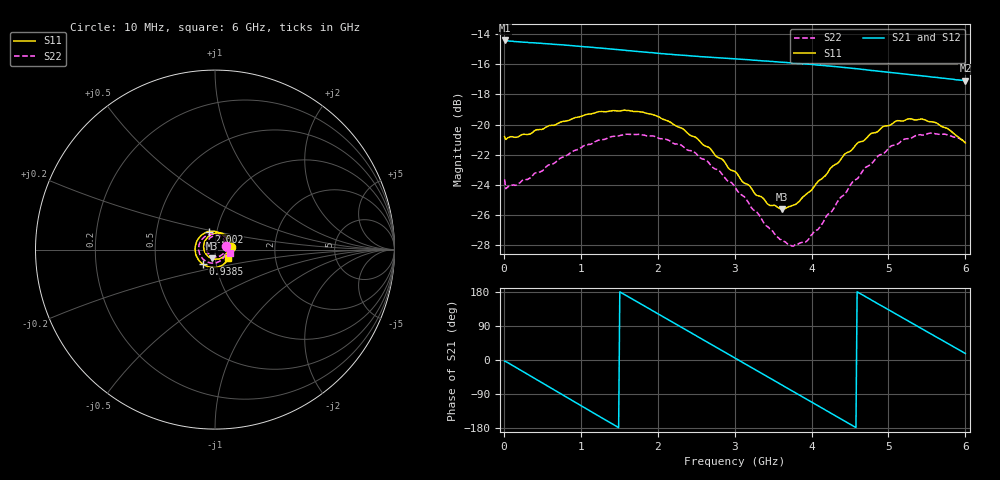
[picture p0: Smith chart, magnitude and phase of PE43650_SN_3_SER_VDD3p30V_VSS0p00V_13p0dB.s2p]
!Keysight Technologies,N5245B,MY57181451,A.13.50.07
!Date: Tuesday, May 07, 2019 08:00:11
!Correction: S11(Full 2 Port(1,2))
!S21(Full 2 Port(1,2))
!S12(Full 2 Port(1,2))
!S22(Full 2 Port(1,2))
!S2P File: Measurements: S11, S21, S12, S22:
# Hz S  dB  R 50
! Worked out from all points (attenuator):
!   401 points, 10 MHz to 6 GHz, reference 50 ohm
!   highest |S21| = -14.42 dB at 10 MHz (marker M1); lowest = -17.1 dB at 6 GHz (marker M2)
!   lowest |S11| = -25.6 dB at 3.619 GHz (marker M3), VSWR 1.11, Z = 47.9 - j4.67 ohm
!   |S11| at or under -10 dB: start of sweep to end of sweep
!   |S22| runs from -28.1 to -20.6 dB; largest |S21 - S12| = 0.0014
!   S11 on the Smith chart (normalised r, x): 10 MHz: 1.20, +0.03; 938.5 MHz: 0.86, -0.14; 2.002 GHz: 0.92, +0.19; 6 GHz: 1.15, -0.11
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1e7  -20.81 9.0  -14.42 -3.3  -14.48 -3.4  -23.64 16.9
2.496e8  -20.66 -37.1  -14.54 -30.7  -14.58 -30.7  -23.69 -36.8
5.1915e8  -20.28 -75.2  -14.63 -63.0  -14.67 -63.0  -22.98 -75.5
9.3845e8  -19.53 -129.5  -14.79 -113.0  -14.84 -113.0  -21.70 -127.6
1.013325e9  -19.45 -138.8  -14.82 -121.8  -14.87 -121.9  -21.50 -136.6
1.2679e9  -19.14 -168.7  -14.93 -152.0  -14.99 -151.9  -21.02 -164.6
1.492525e9  -19.10 165.3  -15.03 -178.4  -15.10 -178.4  -20.76 171.4
1.732125e9  -19.13 138.5  -15.15 153.5  -15.21 153.5  -20.66 146.6
2.001675e9  -19.47 109.0  -15.27 122.0  -15.33 122.0  -20.89 119.5
2.01665e9  -19.50 107.3  -15.28 120.2  -15.33 120.3  -20.91 117.9
2.241275e9  -20.10 82.1  -15.37 94.0  -15.43 94.1  -21.29 94.7
2.4659e9  -20.80 56.1  -15.46 67.9  -15.51 67.9  -21.79 71.7
2.750425e9  -22.06 22.5  -15.56 34.8  -15.61 34.8  -22.96 40.7
3.005e9  -23.12 -11.8  -15.64 5.1  -15.70 5.2  -24.15 11.4
3.289525e9  -24.72 -54.8  -15.75 -28.1  -15.79 -28.0  -25.82 -27.6
3.618975e9  -25.62 -111.8  -15.87 -66.5  -15.92 -66.5  -27.70 -81.1
3.7837e9  -25.32 -141.4  -15.93 -85.7  -15.98 -85.7  -27.98 -111.6
4.008325e9  -24.31 -178.6  -16.01 -111.9  -16.08 -111.9  -27.30 -152.8
4.517475e9  -21.73 112.9  -16.26 -171.4  -16.31 -171.3  -23.92 132.4
5.01165e9  -20.06 59.2  -16.54 131.3  -16.59 131.4  -21.53 78.0
5.475875e9  -19.69 14.4  -16.79 77.6  -16.84 77.7  -20.68 33.7
6e9  -21.22 -31.6  -17.09 17.2  -17.14 17.3  -21.18 -11.7
